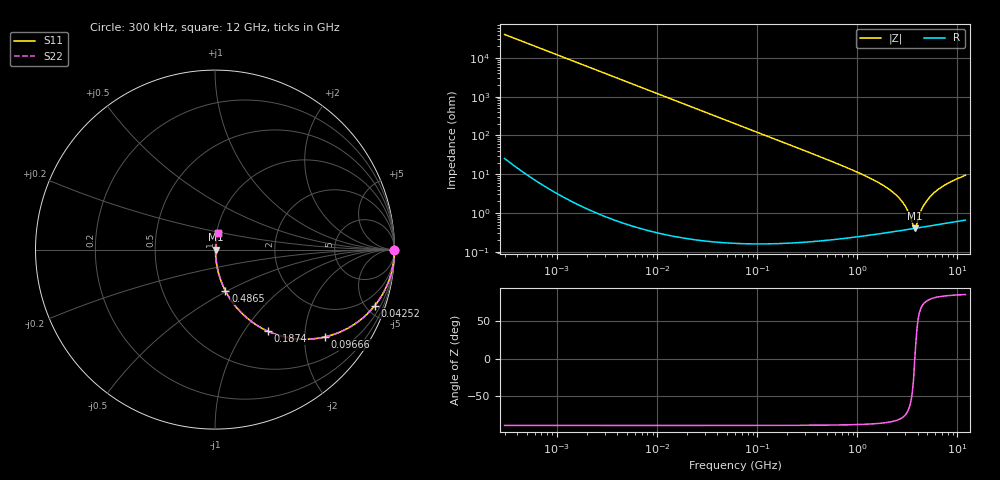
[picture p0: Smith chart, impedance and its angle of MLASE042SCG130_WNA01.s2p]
! MLASE042SCG130_WNA01  S-PARAMETER MODEL  ( General Type )
! Model Generated by TAIYO YUDEN Corporation (http://www.ty-top.com)
! Version 1.0
! TAIYO YUDEN Control No. 130801
! Copyright(c) 2013 TAIYO YUDEN CO.,LTD. All Rights Reserved.
! Product Description (link to TY-COMPAS)
! https://ds.yuden.co.jp/TYCOMPAS/or/detail?pn=MLASE042SCG130JWNA01&u=M
! Products Name : Multilayer Ceramic Capacitors
! Characteristics :
!  Capacitance : 13 pF , Rated Voltage : 16V , TCC : CG / C0G
!  Case Size : 0.4 x 0.2 / 0.016 x 0.008 [mm/inch] , Thickness : 0.2 / 0.008 [mm/inch]
!  (Conditions: Temperature = 25 degC , DC Bias Current/Voltage = 0A / 0V)
! External Node Assignments :
!  1  o---| |---o  2
! GND o---------o GND
! Frequency Range : 0.3MHz  -  12000MHz  [ 401 STEP ]
# MHz S RI R 50
! Freq[MHz].  S11 Real  S11 Imag  S21 Real  S21 Imag  S12 Real  S12 Imag  S22 Real  S22 Imag
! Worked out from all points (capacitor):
!   401 points, 300 kHz to 12 GHz, reference 50 ohm
!   read as one part in series: C = 13.1 pF near 316.3 kHz
!   lowest |Z| = 400 mohm at 3.741 GHz (marker M1)
!   series resonance near 3.75 GHz, so ESL is about 140 pH
!   S11 on the Smith chart (normalised r, x): 300 kHz: open; 42.52 MHz: 1.00, -5.70; 96.66 MHz: 1.00, -2.51; 187.4 MHz: 1.00, -1.29; 486.5 MHz: 1.00, -0.49; 12 GHz: 1.01, +0.19
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0.3  1 -0.00248  7.68e-06 0.00248  7.68e-06 0.00248  1 -0.00248
1.769972  0.9998 -0.0146  0.000216 0.0146  0.000216 0.0146  0.9998 -0.0146
10.44266  0.9926 -0.0855  0.00739 0.0855  0.00739 0.0855  0.9926 -0.0855
23.73947  0.963 -0.1886  0.037 0.1886  0.037 0.1886  0.963 -0.1886
42.51912  0.8902 -0.3123  0.1098 0.3123  0.1098 0.3123  0.8902 -0.3123
60  0.8028 -0.3975  0.1972 0.3975  0.1972 0.3975  0.8028 -0.3975
96.65937  0.6107 -0.487  0.3893 0.487  0.3893 0.487  0.6107 -0.487
187.4445  0.2942 -0.4544  0.7058 0.4544  0.7058 0.4544  0.2942 -0.4544
353.9943  0.1045 -0.3033  0.8955 0.3033  0.8955 0.3033  0.1045 -0.3033
486.4723  0.0582 -0.2302  0.9418 0.2302  0.9418 0.2302  0.0582 -0.2302
1197.383  0.0107 -0.0898  0.9893 0.0898  0.9893 0.0898  0.0107 -0.0898
2088.533  0.00474 -0.0399  0.9953 0.0399  0.9953 0.0399  0.00474 -0.0399
2870.14  0.00388 -0.0176  0.9961 0.0176  0.9961 0.0176  0.00388 -0.0176
3190.978  0.00384 -0.0106  0.9962 0.0106  0.9962 0.0106  0.00384 -0.0106
3547.679  0.00391 -0.00381  0.9961 0.00381  0.9961 0.00381  0.00391 -0.00381
3740.715  0.00398 -0.000147  0.996 0.000147  0.996 0.000147  0.00398 -0.000147
3944.255  0.00408 0.00347  0.9959 -0.00347  0.9959 -0.00347  0.00408 0.00347
4270.516  0.00429 0.00949  0.9957 -0.00949  0.9957 -0.00949  0.00429 0.00949
4623.766  0.00458 0.0153  0.9954 -0.0153  0.9954 -0.0153  0.00458 0.0153
5715.274  0.0057 0.0308  0.9943 -0.0308  0.9943 -0.0308  0.0057 0.0308
7854.144  0.00854 0.0555  0.9915 -0.0555  0.9915 -0.0555  0.00854 0.0555
12000  0.015 0.0917  0.985 -0.0917  0.985 -0.0917  0.015 0.0917
